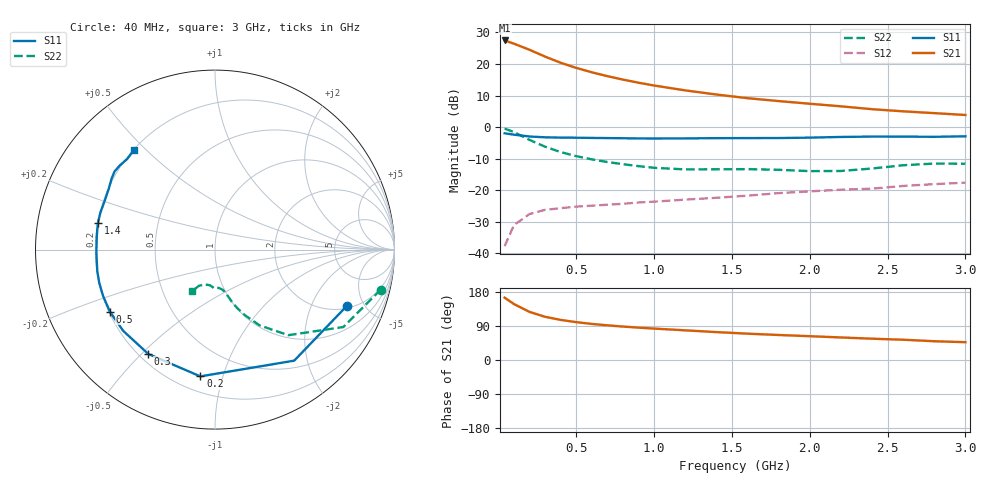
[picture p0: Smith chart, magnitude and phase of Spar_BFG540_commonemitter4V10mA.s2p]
! Filename:  BFG540B.S2P  Version:  3.0
! NXP part #: BFG540  Date: Feb 1992
! Bias condition: Vce=4V, Ic=10mA
! IN LINE PINNING: same data as with cross emitter pinning.
#  MHz  S  MA  R  50
! Freq  S11  S21  S12  S22  !GUM [dB]
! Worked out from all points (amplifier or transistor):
!   21 points, 40 MHz to 3 GHz, reference 50 ohm
!   highest |S21| = 27.5 dB at 40 MHz (marker M1)
!   |S21| within 3 dB of that: start of sweep to 202.3 MHz
!   unconditionally stable (mu >= 1): 1.191 GHz to end of sweep
!   at 300 MHz: K = 0.32, MSG = 24.3 dB, |S12| = -26.2 dB
!   at 1 GHz: K = 0.90, MSG = 18.4 dB, |S12| = -23.6 dB
!   at 3 GHz: K = 1.23, MAG = 7.8 dB, |S12| = -17.6 dB
!   lowest NFmin = 1.30 dB at 900 MHz
!   S11 on the Smith chart (normalised r, x): 40 MHz: 2.15, -3.72; 200 MHz: 0.30, -0.85; 300 MHz: 0.24, -0.52; 500 MHz: 0.20, -0.26; 1.4 GHz: 0.20, +0.11; 3 GHz: 0.20, +0.46
40  0.799 -23.1  23.64 164.6  0.013 77.3  0.95 -13.6
100  0.76 -54.5  21.01 147.6  0.028 61.7  0.835 -31.1
200  0.711 -96.6  16.83 126.9  0.042 47.0  0.628 -49.4
300  0.69 -122.6  13.11 114.0  0.049 39.9  0.49 -59.5
400  0.683 -138.5  10.48 105.8  0.052 37.6  0.403 -65.4
500  0.68 -149.5  8.682 99.9  0.055 36.6  0.347 -69.3
600  0.675 -157.5  7.399 95.2  0.057 37.0  0.309 -71.9
700  0.671 -163.9  6.429 91.5  0.059 38.0  0.28 -73.7
800  0.667 -169.4  5.671 88.2  0.061 39.1  0.259 -75.3
900  0.662 -174.3  5.06 85.4  0.064 40.7  0.241 -77.2
1000  0.661 -178.9  4.569 82.9  0.066 42.4  0.227 -79.4
1200  0.663 173.4  3.823 78.3  0.071 45.6  0.214 -84.7
1400  0.669 167.3  3.288 73.6  0.076 47.6  0.215 -89.1
1600  0.671 161.9  2.878 69.5  0.082 51.0  0.216 -91.2
1800  0.672 156.1  2.589 66.0  0.09 52.6  0.211 -92.9
2000  0.682 150.2  2.349 62.8  0.096 54.9  0.201 -97.9
2200  0.699 145.5  2.138 59.5  0.102 56.4  0.202 -106.6
2400  0.709 142.1  1.926 56.2  0.106 58.3  0.221 -114.1
2600  0.708 138.6  1.78 53.5  0.117 59.0  0.249 -117.2
2800  0.703 134.1  1.667 49.5  0.125 58.1  0.265 -117.5
3000  0.716 128.9  1.558 47.0  0.132 59.9  0.263 -119.1
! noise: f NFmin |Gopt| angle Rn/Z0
900  1.3  0.298  143  0.1
2000  2.1  0.537  -162  0.09
